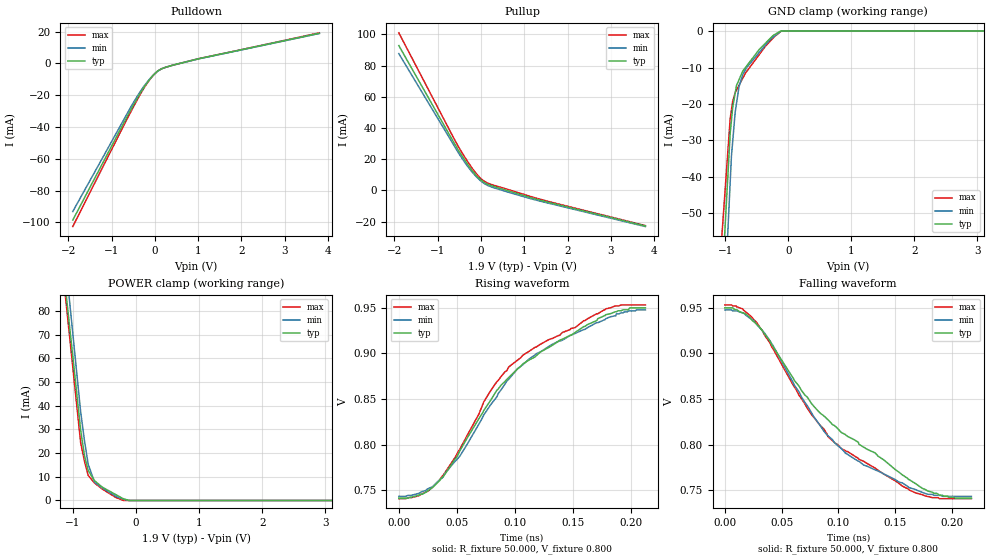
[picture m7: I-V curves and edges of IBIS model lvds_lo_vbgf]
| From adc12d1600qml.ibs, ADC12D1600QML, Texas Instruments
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[Model]   lvds_lo_vbgf
Model_type Output
Vref=0.80E+00
Rref=5.000E+01
Cref=0.000E+00
Vmeas=0.80E+00
C_comp   4.84E-13   4.84E-13   4.84E-13
[Voltage Range]   1.900E+00   1.800E+00   2.000E+00
[POWER Clamp Reference]   1.900E+00   1.800E+00   2.000E+00
[GND Clamp Reference]   0.000E+00   0.000E+00   0.000E+00
[Pullup Reference]   1.900E+00   1.800E+00   2.000E+00
[Pulldown Reference]   0.000E+00   0.000E+00   0.000E+00
[Temperature Range]   25   85   -40
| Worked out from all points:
|   slope of the pulldown table from 0 to 0.285 V, typ, clamps not added: 66.9 ohm
|   slope of the pullup table from 0 to 0.285 V, typ, clamps not added: 70.8 ohm
|   GND clamp passes 1 mA (typ) near -0.22 V on its own axis
|   POWER clamp passes 1 mA (typ) near -0.22 V on its own axis
|   rising waveform, R_fixture 50.000, V_fixture 0.800: 20-80 % time 83.6ps typ, 77.8ps min, 75.9ps max; typ from 0.741 V to 0.95 V
|   falling waveform, R_fixture 50.000, V_fixture 0.800: 20-80 % time 98.4ps typ, 71.4ps min, 79.4ps max; typ from 0.95 V to 0.741 V
[GND Clamp]
-2V       -371.3mA   -433.9mA   -287.7mA
-1.8V     -307.7mA   -361.3mA   -238.9mA
-920mV    -28.13mA   -41.62mA   -24.12mA
-900mV    -24.54mA   -34.36mA   -21.71mA
-880mV    -20.95mA   -30.31mA   -19.3mA
-840mV    -16.96mA   -22.2mA    -16.87mA
-820mV    -14.96mA   -19.9mA    -16.21mA
-780mV    -13.37mA   -15.3mA    -14.89mA
-720mV    -10.98mA   -11.92mA   -12.92mA
-460mV    -5.066mA   -5.895mA   -6.477mA
-120mV    0A         -127.4uA   -143.4uA
4V        0A         0A         0A
[POWER Clamp]
-2.1V     334mA      361.6mA    336.6mA
-1.7V     234.3mA    255.3mA    234.3mA
-980mV    54.74mA    64.08mA    50.07mA
-880mV    29.81mA    37.52mA    24.48mA
-820mV    19.04mA    25.42mA    16.7mA
-760mV    12.67mA    15.24mA    10.56mA
-660mV    8.358mA    7.751mA    7.391mA
-540mV    5.673mA    5.362mA    4.884mA
-320mV    2.445mA    1.745mA    1.257mA
-200mV    684.9uA    507.8uA    0A
-100mV    0A         0A         0A
3.9V      0A         0A         0A
[Pullup]
-1.9V     92.82mA    87.68mA    101mA
-500mV    24.73mA    23.12mA    26.95mA
-220mV    13.23mA    12.23mA    14.78mA
-100mV    9.243mA    8.547mA    10.42mA
60mV      5.314mA    4.666mA    6.188mA
260mV     2.794mA    1.998mA    3.596mA
1.14V     -4.6mA     -5.285mA   -3.869mA
3.8V      -22.85mA   -23.22mA   -22.58mA
[Pulldown]
-1.9V     -98.51mA   -93.11mA   -102.6mA
-700mV    -36.29mA   -34.3mA    -37.8mA
-480mV    -25.22mA   -23.75mA   -26.35mA
-240mV    -14.38mA   -13.75mA   -14.81mA
-40mV     -7.368mA   -7.302mA   -7.39mA
60mV      -4.874mA   -4.928mA   -4.835mA
260mV     -2.27mA    -2.272mA   -2.281mA
1V        2.931mA    2.834mA    2.969mA
3.8V      19mA       18.87mA    19.29mA
[Rising Waveform]
R_fixture = 50.000
V_fixture = 0.800
V_fixture_min = 0.800
V_fixture_max = 0.800
|  time   V(typ)   V(min)   V(max)
0s        741.1mV    743.2mV    740.6mV
17.5ps    744.4mV    746.4mV    743.8mV
35.25ps   760.5mV    761.4mV    761.1mV
52.5ps    792.9mV    787.1mV    794.6mV
79.25ps   848.9mV    843.9mV    859.4mV
94.75ps   873.6mV    871.7mV    885.3mV
107ps     888.7mV    887.8mV    898.2mV
132.5ps   909.2mV    910.3mV    916.6mV
178.3ps   942.6mV    938.1mV    949mV
212.5ps   950.1mV    947.8mV    953.3mV
[Falling Waveform]
R_fixture = 50.000
V_fixture = 0.800
V_fixture_min = 0.800
V_fixture_max = 0.800
|  time   V(typ)   V(min)   V(max)
0s        950.1mV    947.8mV    953.3mV
15.75ps   944.7mV    944.6mV    949mV
27.5ps    932.9mV    932.8mV    935mV
35.25ps   921mV      922.1mV    919.8mV
76.75ps   844.6mV    834.2mV    832.4mV
91ps      827.3mV    809.6mV    808.6mV
106.2ps   811.2mV    790.3mV    793.5mV
168ps     757.3mV    750.7mV    747.1mV
189.2ps   744.4mV    744.3mV    740.6mV
217.5ps   741.1mV    743.2mV    740.6mV
[Ramp]
dV/dt_r   1.7618E+00/8.3350E-11   1.7021E+00/7.6620E-11   1.8224E+00/7.5960E-11
dV/dt_f   1.7618E+00/9.8234E-11   1.7021E+00/7.0641E-11   1.8224E+00/7.9406E-11
R_load = 50
